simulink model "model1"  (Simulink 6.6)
settings: Solver=VariableStepDiscrete  StartTime=0.0  StopTime=0.0  RelTol=1e-3
libraries: ltpda_library x1

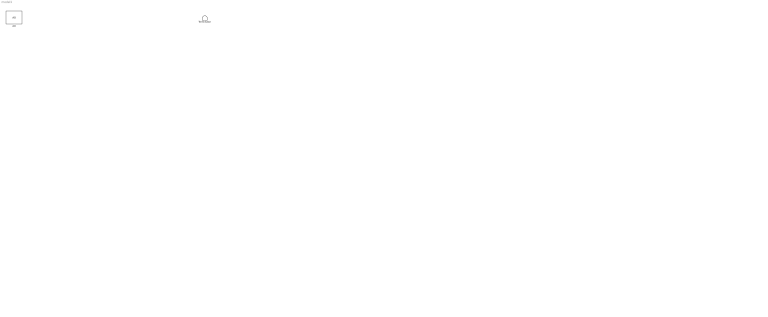
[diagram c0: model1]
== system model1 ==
  note: .
  AO : ltpda_library/AO  Tag=input  SystemSampleTime=-1
  Terminator : Terminator
